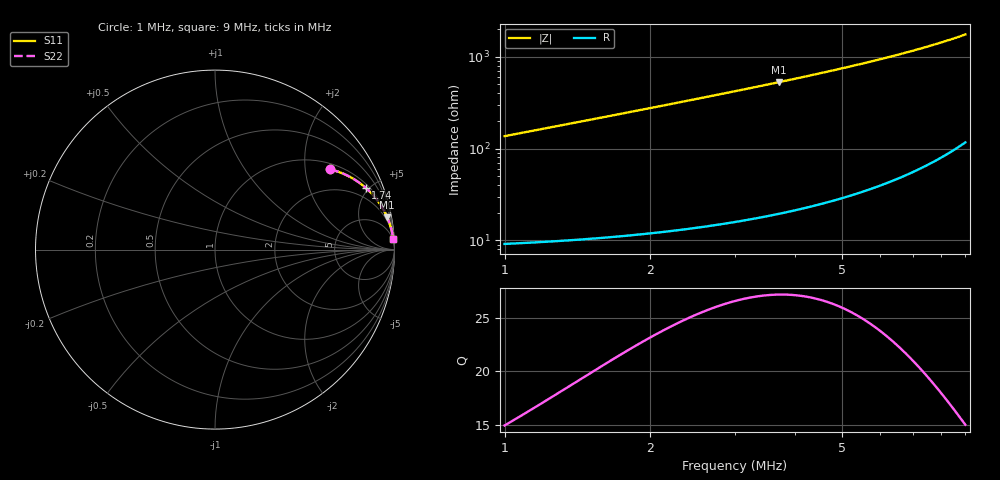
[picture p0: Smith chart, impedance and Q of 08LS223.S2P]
! Coilcraft 0805LS-223 Chip Inductor
! 18 September 2002
# MHZ S MA R 50
!Freq  MagS11  AngS11  MagS21  AngS21  MagS12  AngS12  MagS22  AngS22
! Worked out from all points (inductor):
!   401 points, 1 MHz to 9 MHz, reference 50 ohm
!   read as one part in series: L = 21.8 uH near 1.04 MHz
!   highest Q = 27.2 at 3.7 MHz (marker M1), where L = 22.8 uH
!   S11 on the Smith chart (normalised r, x): 1 MHz: 1.18, +2.72; 1.74 MHz: 1.22, +4.78; 9 MHz: 3, +35
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1  0.7822 34.9  0.5729 -51.3  0.5729 -51.3  0.7822 34.9
1.04  0.7937 33.9  0.5589 -52.4  0.5589 -52.4  0.7937 33.9
1.12  0.8144 32.1  0.5323 -54.4  0.5323 -54.4  0.8144 32.1
1.2  0.8324 30.4  0.5076 -56.2  0.5076 -56.2  0.8324 30.4
1.28  0.8481 28.9  0.4845 -57.9  0.4845 -57.9  0.8481 28.9
1.36  0.8618 27.5  0.4631 -59.4  0.4631 -59.4  0.8618 27.5
1.54  0.8869 24.8  0.4201 -62.3  0.4201 -62.3  0.8869 24.8
1.74  0.9077 22.3  0.3797 -65.1  0.3797 -65.1  0.9077 22.3
1.88  0.9191 20.8  0.3552 -66.7  0.3552 -66.7  0.9191 20.8
2.02  0.9286 19.5  0.3333 -68.1  0.3333 -68.1  0.9286 19.5
2.34  0.945 16.9  0.2913 -70.8  0.2913 -70.8  0.945 16.9
2.62  0.9551 15.2  0.2616 -72.6  0.2616 -72.6  0.9551 15.2
2.92  0.9631 13.6  0.2352 -74.2  0.2352 -74.2  0.9631 13.6
3.28  0.9702 12.1  0.2091 -75.8  0.2091 -75.8  0.9702 12.1
3.68  0.9759 10.7  0.1854 -77.2  0.1854 -77.2  0.9759 10.7
3.7  0.9761 10.6  0.1843 -77.3  0.1843 -77.3  0.9761 10.6
4.32  0.982 9.0  0.1557 -78.9  0.1557 -78.9  0.982 9.0
5  0.9862 7.6  0.1317 -80.2  0.1317 -80.2  0.9862 7.6
5.62  0.9888 6.6  0.1143 -81.1  0.1143 -81.1  0.9888 6.6
6.34  0.9909 5.6  0.09781 -81.9  0.09781 -81.9  0.9909 5.6
7.68  0.9933 4.3  0.07425 -82.7  0.07425 -82.7  0.9933 4.3
9  0.9946 3.2  0.05676 -82.9  0.05676 -82.9  0.9946 3.2
